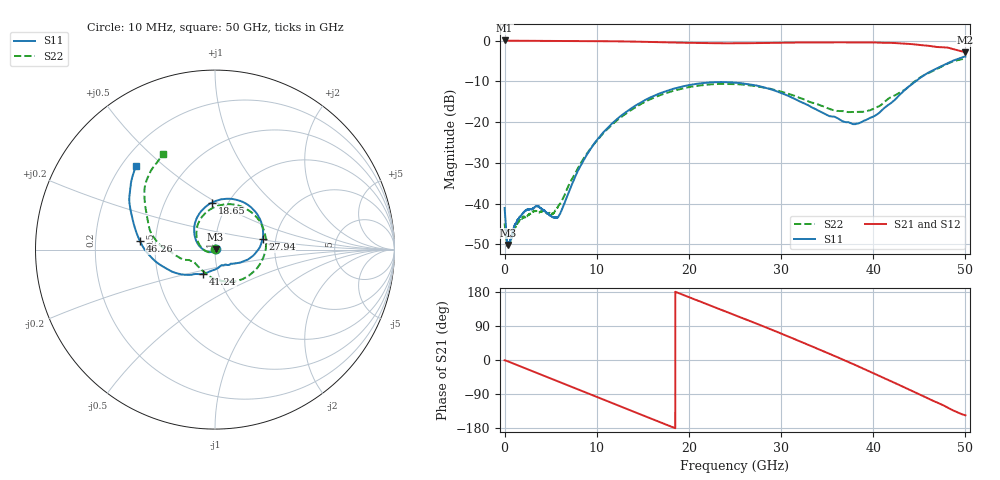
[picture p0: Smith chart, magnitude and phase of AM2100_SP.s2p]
!Keysight Technologies,N5245B,MY58422270,A.16.20.02
!Date: Wednesday, March 11, 2026 22:59:50
!Correction: S11(C  2-Port  )
!S21(C  2-Port  )
!S12(C  2-Port  )
!S22(C  2-Port  )
!S2P File: Measurements: S11, S21, S12, S22:
# Hz S  dB  R 50
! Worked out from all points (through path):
!   6401 points, 10 MHz to 50 GHz, reference 50 ohm
!   highest |S21| = 0.05 dB at 10 MHz (marker M1); lowest = -2.8 dB at 50 GHz (marker M2)
!   group delay of S21, straight-line fit = 27.8 ps
!   lowest |S11| = -50.2 dB at 353.7 MHz (marker M3), VSWR 1.01, Z = 50.3 + j0.0656 ohm
!   |S11| at or under -10 dB: start of sweep to 44.59 GHz
!   |S22| runs from -50.5 to -4.4 dB; largest |S21 - S12| = 0.013
!   S11 on the Smith chart (normalised r, x): 10 MHz: 1.02, +0.01; 18.65 GHz: 0.84, +0.48; 27.94 GHz: 1.70, +0.21; 41.24 GHz: 0.85, -0.23; 46.26 GHz: 0.41, +0.05; 50 GHz: 0.26, +0.41
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1e7  -41.09 29.4  0.05 -0.9  -0.06 -1.0  -44.88 97.9
3.536812e8  -50.17 12.1  -0.01 -3.5  -0.01 -3.5  -50.24 76.5
5.489547e8  -49.45 61.4  -0.01 -5.4  -0.01 -5.4  -49.83 -12.7
1.501889e9  -43.78 51.7  -0.02 -14.6  -0.02 -14.6  -44.50 49.3
2.407958e9  -41.56 43.0  -0.03 -23.4  -0.03 -23.4  -43.03 30.2
5.829148e9  -43.30 -62.6  -0.06 -56.5  -0.06 -56.5  -40.64 -79.0
8.34427e9  -30.37 -153.3  -0.08 -81.0  -0.08 -81.0  -29.81 -150.6
1.214039e10  -19.40 158.6  -0.16 -118.1  -0.16 -118.1  -19.70 156.1
1.667854e10  -13.10 112.3  -0.37 -162.2  -0.37 -162.2  -13.55 104.9
1.865471e10  -11.61 93.6  -0.47 178.8  -0.47 178.7  -12.11 84.2
2.167754e10  -10.39 66.2  -0.60 150.0  -0.60 150.1  -10.90 52.9
2.5005e10  -10.32 37.1  -0.63 118.5  -0.63 118.5  -10.69 18.6
2.794191e10  -11.35 12.1  -0.58 90.1  -0.58 90.2  -11.43 -13.3
3.060544e10  -13.39 -9.4  -0.49 63.9  -0.50 63.8  -12.90 -45.7
3.333927e10  -16.39 -29.0  -0.44 36.0  -0.44 36.0  -15.21 -81.3
3.744001e10  -20.15 -62.3  -0.40 -6.6  -0.40 -6.6  -17.52 -133.6
4.124394e10  -16.46 -116.0  -0.52 -48.0  -0.52 -48.0  -14.98 -161.5
4.167354e10  -15.74 -123.3  -0.53 -52.7  -0.54 -52.7  -14.20 -165.2
4.389966e10  -11.21 -154.6  -0.80 -78.4  -0.81 -78.3  -11.19 179.4
4.625856e10  -7.51 173.4  -1.33 -104.9  -1.33 -104.9  -7.68 155.7
4.839876e10  -5.16 149.9  -1.87 -129.8  -1.88 -129.6  -5.33 134.9
5e10  -3.89 133.3  -2.82 -146.0  -2.85 -145.8  -4.36 118.8
